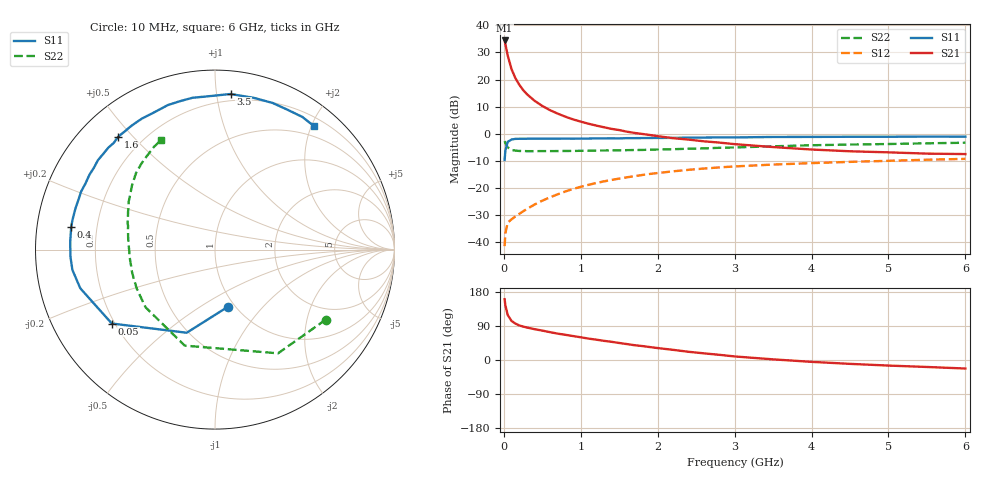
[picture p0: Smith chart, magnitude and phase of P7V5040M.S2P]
! SIEMENS Small Signal Semiconductors
! BFP196
! Si NPN RF Bipolar Junction Transistor in SOT143
! VCE = 0.5 V  IC = 40 mA
! Common Emitter S-Parameters:  May  1996
# GHz  S  MA  R  50
!  f  S11  S21  S12  S22
! GHz  MAG  ANG  MAG  ANG  MAG  ANG  MAG  ANG
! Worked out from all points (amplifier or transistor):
!   36 points, 10 MHz to 6 GHz, reference 50 ohm
!   highest |S21| = 34.4 dB at 10 MHz (marker M1)
!   |S21| within 3 dB of that: start of sweep to 31.79 MHz
!   unconditionally stable (mu >= 1): 348.9 MHz to end of sweep
!   at 250 MHz: K = 0.89, MSG = 22.4 dB, |S12| = -28.7 dB
!   at 1.4 GHz: K = 1.16, MAG = 7.0 dB, |S12| = -17.1 dB
!   at 6 GHz: K = 1.05, MAG = -0.5 dB, |S12| = -9.3 dB
!   S11 on the Smith chart (normalised r, x): 10 MHz: 0.93, -0.66; 50 MHz: 0.19, -0.31; 400 MHz: 0.10, +0.08; 1.6 GHz: 0.11, +0.46; 3.5 GHz: 0.15, +1.09; 6 GHz: 0.33, +2.05
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0.01  0.3266 -77.3  52.66 160.4  0.0084 69.6  0.7301 -32.3
0.02  0.4894 -108.8  45.03 144.2  0.0146 58.0  0.6763 -58.7
0.05  0.7073 -144.4  27.84 118.8  0.0228 39.8  0.5609 -107.5
0.1  0.781 -164.0  15.54 103.1  0.0263 37.3  0.5031 -140.2
0.15  0.8025 -171.9  10.63 96.1  0.0298 39.6  0.4874 -153.2
0.2  0.8061 -177.0  8.044 91.3  0.0331 43.4  0.4807 -160.4
0.25  0.8065 179.2  6.425 88.2  0.0369 47.1  0.4789 -165.3
0.3  0.808 176.5  5.37 85.7  0.0409 50.0  0.4764 -168.2
0.4  0.811 171.1  4.052 81.3  0.0493 53.7  0.4766 -172.7
0.5  0.811 168.1  3.253 77.6  0.0581 56.1  0.4775 -175.9
0.6  0.8106 163.5  2.722 73.5  0.067 57.4  0.4771 -178.1
0.7  0.8099 159.8  2.349 69.6  0.0761 57.8  0.4785 179.9
0.9  0.8102 153.0  1.839 63.2  0.0955 57.1  0.4808 176.6
1.1  0.8142 146.0  1.53 56.5  0.1139 55.5  0.4864 173.8
1.3  0.8199 139.3  1.317 50.6  0.1318 52.9  0.4901 171.0
1.6  0.8286 130.6  1.09 42.0  0.1569 48.8  0.4973 167.3
2.2  0.8366 113.8  0.828 26.8  0.2022 39.5  0.5177 159.5
3  0.8541 93.9  0.642 9.4  0.2489 26.9  0.5581 148.4
3.5  0.8712 84.3  0.567 1.7  0.2696 20.0  0.5855 142.1
4.5  0.8778 68.5  0.474 -10.2  0.3023 7.8  0.6308 130.5
5.5  0.8849 56.6  0.429 -18.4  0.3309 -2.9  0.6652 120.9
6  0.8819 51.1  0.421 -22.5  0.3435 -8.6  0.6817 116.0
